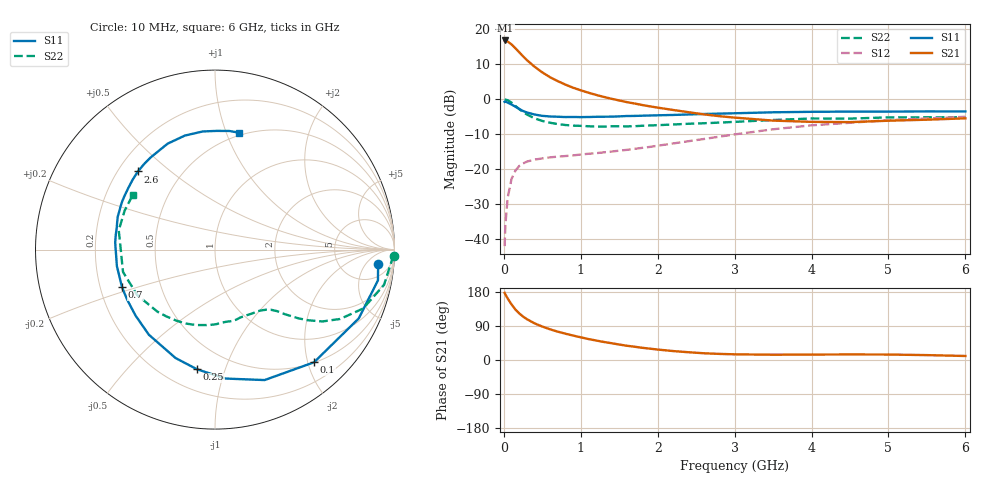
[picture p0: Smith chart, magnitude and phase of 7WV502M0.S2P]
! Infineon Technologies  Discrete & RF Semiconductors
! BFS17W
! Si NPN RF Bipolar Junction Transistor in SOT323
! VCE = 0.5 V  IC = 2 mA
! Common Emitter S-Parameters:  August  1999
# GHz  S  MA  R  50
!  f  S11  S21  S12  S22
! GHz  MAG  ANG  MAG  ANG  MAG  ANG  MAG  ANG
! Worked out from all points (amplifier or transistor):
!   36 points, 10 MHz to 6 GHz, reference 50 ohm
!   highest |S21| = 16.7 dB at 20 MHz (marker M1)
!   |S21| within 3 dB of that: start of sweep to 184 MHz
!   unconditionally stable (mu >= 1): 706.8 MHz to end of sweep
!   at 250 MHz: K = 0.41, MSG = 15.3 dB, |S12| = -18.4 dB
!   at 1.4 GHz: K = 1.46, MAG = 3.5 dB, |S12| = -15.0 dB
!   at 6 GHz: K = 1.16, MAG = -2.6 dB, |S12| = -5.1 dB
!   S11 on the Smith chart (normalised r, x): 10 MHz: 11, -11; 100 MHz: 0.51, -2.11; 250 MHz: 0.33, -0.80; 700 MHz: 0.29, -0.18; 2.6 GHz: 0.28, +0.39; 6 GHz: 0.48, +1.11
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0.01  0.9125 -5.1  6.823 177.1  0.0079 84.5  0.9951 -1.9
0.02  0.9239 -10.7  6.874 172.9  0.0159 85.8  0.9816 -4.8
0.05  0.8879 -25.6  6.628 162.2  0.039 75.9  0.962 -11.8
0.1  0.8358 -48.7  6.029 146.7  0.0722 62.9  0.8881 -21.7
0.15  0.7776 -69.2  5.323 133.3  0.0947 53.0  0.7971 -29.0
0.2  0.7207 -85.4  4.666 123.0  0.1106 46.3  0.7198 -33.8
0.25  0.674 -98.6  4.079 114.6  0.12 40.6  0.6512 -37.2
0.3  0.6429 -110.0  3.599 107.7  0.1277 37.6  0.602 -39.5
0.4  0.6007 -127.8  2.894 96.6  0.1366 32.9  0.5291 -42.8
0.5  0.5754 -140.3  2.405 88.3  0.1416 30.9  0.4864 -44.8
0.6  0.5633 -150.2  2.052 81.0  0.1468 29.8  0.4586 -47.0
0.7  0.5589 -158.0  1.805 74.9  0.1503 29.8  0.4393 -49.7
0.9  0.5544 -170.5  1.453 64.5  0.1566 30.5  0.4168 -55.6
1.1  0.5538 179.5  1.231 55.3  0.1652 32.4  0.4085 -62.2
1.3  0.5591 171.3  1.073 47.6  0.1732 34.5  0.4039 -69.8
1.6  0.5722 161.3  0.903 37.6  0.1879 37.9  0.4069 -81.1
2.2  0.5924 144.7  0.698 23.6  0.2318 43.5  0.4331 -103.9
2.6  0.6116 134.6  0.604 17.8  0.2686 44.8  0.451 -118.9
3.5  0.6466 114.1  0.492 13.9  0.3697 41.4  0.5019 -149.6
4.5  0.6617 95.9  0.468 14.7  0.4579 31.3  0.5256 179.5
5.5  0.6658 83.1  0.507 12.9  0.5285 21.8  0.5483 156.6
6  0.6649 78.2  0.53 10.6  0.558 17.1  0.5498 146.5
